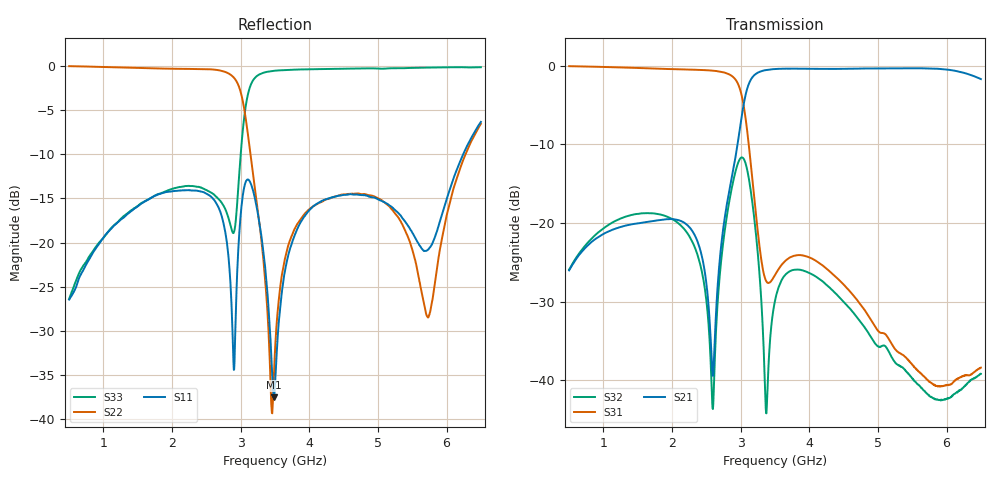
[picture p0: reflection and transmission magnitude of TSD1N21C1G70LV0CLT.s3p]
# MHZ S RI R 50
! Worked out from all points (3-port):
!   1201 points, 500 MHz to 6.5 GHz, reference 50 ohm
!   strongest paths, dB at 500 MHz, 2 GHz, 3.5 GHz, 5 GHz, 6.5 GHz:
!     S21: -26.0, -19.5, -0.4, -0.3, -1.7
!     S31: -0.1, -0.4, -26.6, -33.6, -38.4
!     S32: -25.9, -19.5, -29.9, -35.7, -39.2
!   lowest |S11| = -37.5 dB at 3.485 GHz (marker M1), VSWR 1.03, Z = 50.9 - j1 ohm
!   |S11| at or under -10 dB: start of sweep to 6.242 GHz
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500  -0.0252 -0.0403  0.0139 0.048  0.9369 -0.3314
     0.014 0.0481  0.9074 -0.4169  0.0259 0.0435
     0.9367 -0.3307  0.0257 0.0436  -0.00218 -0.0478
2090  -0.0104 0.1966  0.0693 0.0782  -0.0791 -0.9459
      0.0695 0.0781  -0.1983 -0.944  0.0615 -0.0788
      -0.0785 -0.9458  0.0614 -0.0787  -0.0337 -0.2028
2595  0.1774 -0.00458  -0.00351 0.01  -0.7006 -0.6122
      -0.0036 0.0101  -0.665 -0.6872  0.00604 -0.00251
      -0.7005 -0.612  0.00608 -0.0025  -0.000431 -0.189
2990  0.082 0.0995  -0.4004 0.0586  -0.5484 0.4498
      -0.4003 0.0579  -0.7026 0.2135  0.1409 -0.2124
      -0.5485 0.4492  0.1407 -0.2139  0.2782 0.036
3370  -0.0199 -0.0606  0.00919 0.938  -0.037 0.0215
      0.00903 0.9388  -0.0349 0.0395  0.00171 0.0061
      -0.0371 0.0215  0.00173 0.00595  0.3987 -0.8342
3485  0.00893 -0.00984  0.2359 0.9211  -0.0451 -0.00598
      0.2354 0.9221  -0.002 -0.0178  0.0257 -0.0148
      -0.0451 -0.00611  0.0256 -0.0149  0.246 -0.9073
3500  0.0144 -0.00573  0.2615 0.9152  -0.046 -0.00845
      0.2609 0.9162  0.000821 -0.0246  0.0268 -0.0175
      -0.046 -0.00855  0.0268 -0.0176  0.2285 -0.9134
4900  0.1135 -0.1408  0.9455 -0.1448  -0.0241 -0.00194
      0.9499 -0.1454  -0.15 -0.1074  -0.0162 -0.00978
      -0.0241 -0.002  -0.0161 -0.00973  -0.7285 -0.6414
5730  0.0888 -0.0202  0.6455 -0.7133  -0.00754 0.00653
      0.6439 -0.7143  -0.00277 0.0375  -0.00815 -0.00085
      -0.00754 0.00653  -0.00807 -0.000819  -0.9082 -0.3694
6500  0.4728 0.0967  -0.0691 -0.8209  0.000706 0.0119
      -0.0726 -0.8191  0.3945 -0.2567  -0.0113 0.00072
      0.00051 0.012  -0.011 0.000599  -0.9461 -0.2748
